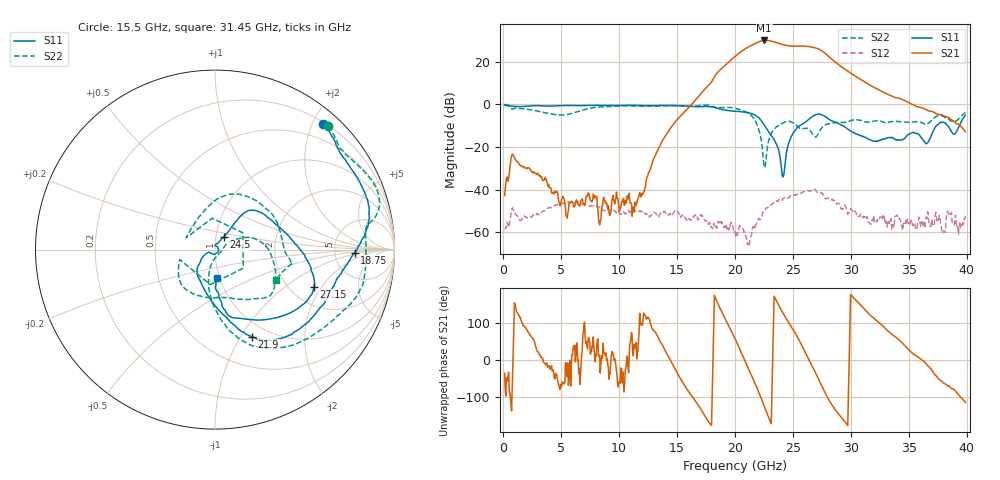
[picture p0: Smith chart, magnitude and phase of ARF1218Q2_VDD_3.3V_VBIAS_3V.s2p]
!Bias:VDD=3.3V, VBIAS=3.0V
# GHz S DB R 50.0
!freq dBS11 angS11 dBS21 angS21 dBS12 angS12 dBS22 angS22
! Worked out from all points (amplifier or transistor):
!   796 points, 150 MHz to 39.9 GHz, reference 50 ohm
!   highest |S21| = 30.0 dB at 22.55 GHz (marker M1)
!   |S21| within 3 dB of that: 21.21 GHz to 26.56 GHz (5.352 GHz wide, 22.4 % of centre)
!   unconditionally stable (mu >= 1): start of sweep to end of sweep
!   at 6.75 GHz: K = 1131.10, MAG = -32.9 dB, |S12| = -46.4 dB
!   at 20.05 GHz: K = 6.61, MAG = 30.4 dB, |S12| = -60.6 dB
!   at 39.9 GHz: K = 364.38, MAG = -8.9 dB, |S12| = -52.3 dB
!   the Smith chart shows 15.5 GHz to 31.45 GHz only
!   S11 on the Smith chart (normalised r, x): 15.5 GHz: 0.23, +2.16; 18.75 GHz: 7.92, -0.72; 21.9 GHz: 0.84, -1.12; 24.5 GHz: 1.09, +0.15; 27.15 GHz: 2.67, -1.70; 31.45 GHz: 0.97, -0.31
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0.15  -0.26 -8.0  -42.77 -35.5  -58.36 53.8  -0.01 -13.5
6.8  -0.58 176.1  -44.56 17.6  -46.53 50.1  -2.84 167.0
13.4  -0.56 80.3  -21.01 61.0  -51.96 -16.7  -0.80 75.2
15.5  -0.70 49.4  -4.55 -58.9  -51.68 -42.7  -0.60 47.5
18.75  -2.19 -1.3  16.18 137.9  -55.39 -60.4  -1.50 0.3
20.05  -3.18 -17.1  22.56 56.0  -60.56 -45.3  -1.79 -21.8
21.1  -3.85 -44.6  26.65 -17.5  -65.79 -6.2  -3.92 -59.8
21.9  -5.57 -66.9  28.93 -72.8  -55.87 81.7  -9.14 -88.2
22.55  -9.58 -87.1  29.99 -123.6  -49.66 45.6  -29.34 -58.5
23  -13.45 -109.4  29.88 -159.4  -47.32 22.0  -15.60 23.1
23.2  -14.94 -122.0  29.65 -102.3  -47.06 1.6  -13.04 16.5
23.35  -16.16 -130.0  29.41 103.0  -46.21 -5.6  -11.95 10.8
23.45  -17.11 -134.1  29.21 168.3  -46.02 -7.9  -11.34 7.1
23.55  -18.18 -136.7  29.04 161.9  -45.80 -7.8  -10.82 3.1
24.5  -21.60 55.2  27.63 108.5  -43.94 -43.2  -8.03 -35.4
25.5  -10.45 46.8  27.38 56.3  -42.05 -78.1  -10.72 -69.6
26.65  -5.91 -5.0  26.90 -14.3  -40.36 -133.4  -13.33 -158.9
27.15  -4.60 -20.6  26.14 -45.5  -41.46 -157.8  -14.31 122.5
28.5  -8.00 -73.2  20.57 -125.2  -45.03 141.6  -8.73 37.5
31.45  -16.03 -86.4  9.78 128.5  -52.61 32.6  -8.37 -26.3
33.3  -15.64 -79.2  4.50 76.0  -54.88 -27.1  -8.32 -56.1
39.9  -5.14 -143.9  -12.86 -114.0  -52.28 7.2  -3.78 -151.4
